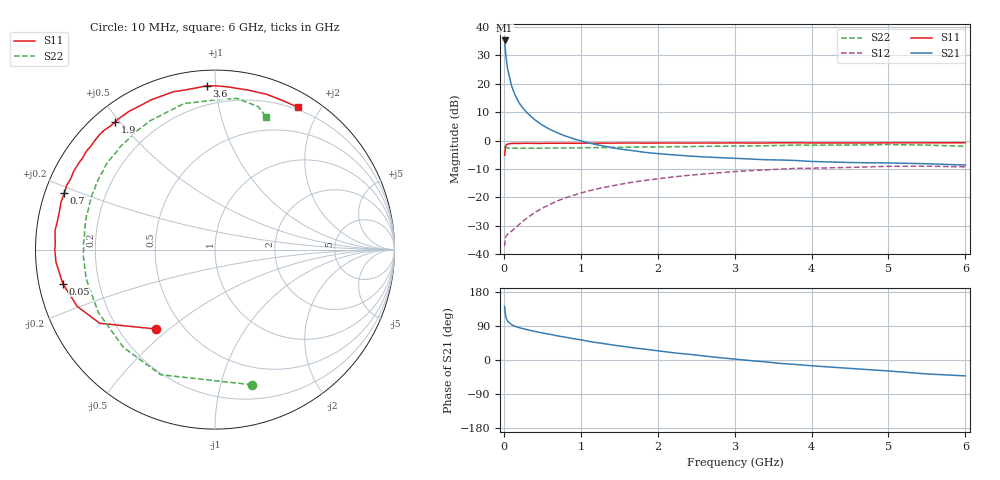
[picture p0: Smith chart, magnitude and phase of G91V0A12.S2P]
! SIEMENS Small Signal Semiconductors
! BFG235
! Si NPN RF Bipolar Junction Transistor in SOT223
! VCE = 1 V  IC = 120 mA
! Common Emitter S-Parameters:  July  1994
# GHz  S  MA  R  50
!  f  S11  S21  S12  S22
! GHz  MAG  ANG  MAG  ANG  MAG  ANG  MAG  ANG
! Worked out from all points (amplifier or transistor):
!   40 points, 10 MHz to 6 GHz, reference 50 ohm
!   highest |S21| = 35.2 dB at 10 MHz (marker M1)
!   |S21| within 3 dB of that: start of sweep to 19 MHz
!   unconditionally stable (mu >= 1): 408.6 MHz to 1.698 GHz; 1.701 GHz to 1.999 GHz
!   at 200 MHz: K = 0.82, MSG = 21.3 dB, |S12| = -29.5 dB
!   at 1.5 GHz: K = 1.02, MAG = 5.4 dB, |S12| = -15.4 dB
!   at 6 GHz: K = 0.95, MSG = 0.3 dB, |S12| = -9.3 dB
!   S11 on the Smith chart (normalised r, x): 10 MHz: 0.35, -0.45; 50 MHz: 0.07, -0.11; 700 MHz: 0.06, +0.18; 1.9 GHz: 0.06, +0.48; 3.6 GHz: 0.09, +0.95; 6 GHz: 0.17, +1.73
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0.01  0.5521 -126.8  57.55 141.1  0.0139 51.1  0.7806 -74.7
0.02  0.7622 -147.4  39.21 121.2  0.0191 35.8  0.7599 -113.4
0.03  0.8303 -157.6  28.41 111.2  0.0209 30.7  0.7464 -133.1
0.05  0.869 -167.4  17.9 101.9  0.0226 26.9  0.7387 -151.6
0.1  0.889 -175.6  9.185 93.3  0.0255 33.3  0.7358 -167.2
0.15  0.8925 -179.9  6.128 88.6  0.029 40.7  0.7324 -173.7
0.2  0.8904 177.7  4.581 85.4  0.0336 45.9  0.7345 -177.4
0.25  0.8941 175.2  3.69 82.5  0.0383 50.2  0.7321 179.9
0.3  0.8974 173.2  3.09 80.3  0.0433 52.9  0.7336 177.5
0.4  0.8916 169.2  2.328 75.5  0.0541 56.2  0.7318 174.0
0.5  0.893 165.8  1.867 71.4  0.0648 57.6  0.7347 170.9
0.7  0.8967 159.5  1.363 63.6  0.0872 57.9  0.7402 165.3
0.9  0.8957 153.8  1.084 56.4  0.1084 55.5  0.7434 160.4
1.1  0.8992 147.6  0.909 49.3  0.1296 52.7  0.7508 155.5
1.5  0.9039 137.9  0.713 37.2  0.1689 45.5  0.7614 146.5
1.9  0.9024 128.2  0.607 26.9  0.2045 38.2  0.7711 138.2
2.2  0.9072 121.8  0.561 19.2  0.2289 32.2  0.7795 132.2
3.2  0.905 100.8  0.474 -1.5  0.2955 12.8  0.8048 113.4
3.6  0.9138 92.9  0.455 -9.1  0.3147 4.6  0.8198 105.4
4.5  0.9077 77.9  0.411 -22.2  0.3378 -10.8  0.8336 90.2
5.5  0.9125 65.2  0.391 -36.8  0.3545 -28.0  0.8321 73.2
6  0.9169 59.8  0.371 -41.9  0.3445 -34.5  0.7924 68.9
